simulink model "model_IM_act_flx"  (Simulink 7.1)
settings: Solver=ode45  StartTime=0.0  StopTime=10.0  RelTol=1e-3

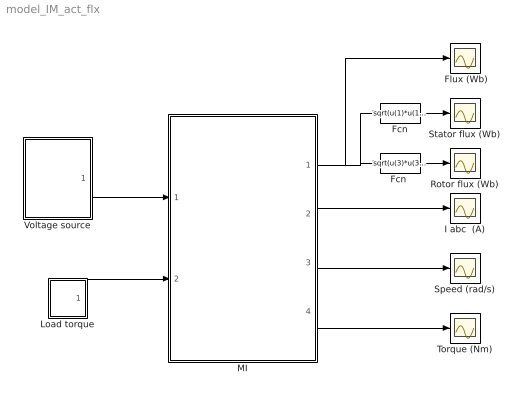
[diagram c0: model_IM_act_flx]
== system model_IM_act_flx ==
  " Flux (Wb)" : Scope
  Fcn : Fcn  Expr=sqrt(u(1)*u(1)+u(2)*u(2))
  "Fcn " : Fcn  Expr=sqrt(u(3)*u(3)+u(4)*u(4))
  I abc  (A) : Scope
  Load torque : Subsystem  mask(Repeating table){}
      mask help: Repeating table. Enter values of time and output for first cycle.
      mask init:
      | period = max(@1); t = @1; y = @2;
  MI : Subsystem  mask(Parameter of induction machine){p=2, Rs=0.3, Rr=0.25, Ls=0.0415, Lr=0.0412, Lm=0.0403, J=0.1, B=0.02}
      mask prompts: p "Poles pairs"; J "Inertial moment"; B "Friction coeficient"
      mask help: The induction machine model in dq frame
      mask init:
      | sigma=1-Lm^2/(Ls*Lr);
      | a11=Rs/(sigma*Ls);
      | a12=Rs*(1-sigma)/(sigma*Lm);
      | a21=Rr*(1-sigma)/(sigma*Lm);
      | a22=Rr/(sigma*Lr);
      | c1=1/(sigma*Ls) ;
      | c2=(sigma-1)/(sigma*Lm);
  Rotor flux (Wb) : Scope
  Speed (rad/s) : Scope
  Stator flux (Wb) : Scope
  Torque (Nm) : Scope
  Voltage source : Subsystem  mask{Vf=220, f1=50}
      mask prompts: Vf "Vf -phase rms value (V)"; f1 "f1 (Hz)"
      mask init:
      | Vm=sqrt(2)*Vf;
      | w1=2*pi*f1;
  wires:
  Fcn/1 -> Stator flux (Wb)/1
  "Fcn "/1 -> Rotor flux (Wb)/1
  MI/1(flux) -> "Fcn "/1, Fcn/1, " Flux (Wb)"/1
  MI/3(w) -> Speed (rad/s)/1
  MI/2("i abc ") -> I abc  (A)/1
  MI/4(Te) -> Torque (Nm)/1
  Voltage source/1(Vabc) -> MI/1(V abc)
  Load torque/1(out_1) -> MI/2(Tload)

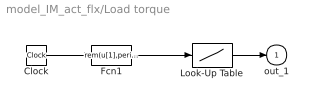
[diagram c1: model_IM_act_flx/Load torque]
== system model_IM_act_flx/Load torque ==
  Clock : Clock
  Fcn1 : Fcn  Expr=rem(u[1],period)
  Look-Up Table : Lookup  InputValues=t  Table=y  OutDataType=sfix(16)  OutScaling=2^0
  out_1 : Outport
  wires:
  Look-Up Table/1 -> out_1/1
  Clock/1 -> Fcn1/1
  Fcn1/1 -> Look-Up Table/1

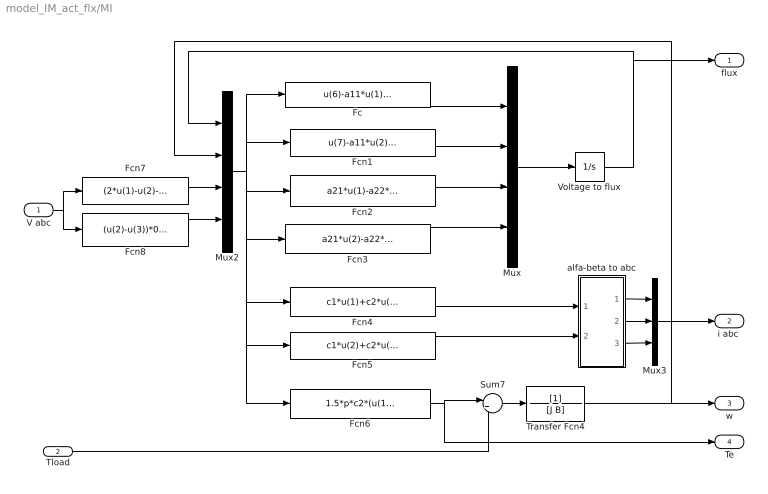
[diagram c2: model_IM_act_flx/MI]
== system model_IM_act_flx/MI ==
  V abc : Inport  OutDataType=sfix(16)  OutScaling=2^0
  Tload : Inport  Port=2  OutDataType=sfix(16)  OutScaling=2^0
  Fc : Fcn  Expr=u(6)-a11*u(1)+a12*u(3)
  Fcn1 : Fcn  Expr=u(7)-a11*u(2)+a12*u(4)
  Fcn2 : Fcn  Expr=a21*u(1)-a22*u(3)-p*u(5)*u(4)
  Fcn3 : Fcn  Expr=a21*u(2)-a22*u(4)+p*u(5)*u(3)
  Fcn4 : Fcn  Expr=c1*u(1)+c2*u(3)
  Fcn5 : Fcn  Expr=c1*u(2)+c2*u(4)
  Fcn6 : Fcn  Expr=1.5*p*c2*(u(1)*u(4)-u(2)*u(3))
  Fcn7 : Fcn  Expr=(2*u(1)-u(2)-u(3))/3
  Fcn8 : Fcn  Expr=(u(2)-u(3))*0.5773502
  Mux : Mux
  Mux2 : Mux
  Mux3 : Mux  Inputs=3
  Sum7 : Sum  Inputs=|+-  OutDataType=sfix(16)  OutScaling=2^0
  Transfer Fcn4 : TransferFcn  Denominator=[J B]
  Voltage to flux : Integrator
  alfa-beta to abc : Subsystem
  flux : Outport
  "i abc " : Outport  Port=2
  w : Outport  Port=3
  Te : Outport  Port=4
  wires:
  Fc/1 -> Mux/1
  Fcn1/1 -> Mux/2
  Fcn2/1 -> Mux/3
  Fcn3/1 -> Mux/4
  Mux2/1 -> Fc/1, Fcn1/1, Fcn2/1, Fcn3/1, Fcn4/1, Fcn6/1, Fcn5/1
  Mux/1 -> Voltage to flux/1
  Voltage to flux/1 -> flux/1, Mux2/1
  Sum7/1 -> Transfer Fcn4/1
  Tload/1 -> Sum7/2
  Fcn6/1 -> Sum7/1, Te/1
  Fcn5/1 -> alfa-beta to abc/2(in_2)
  Transfer Fcn4/1 -> w/1, Mux2/2
  Fcn7/1 -> Mux2/3
  Fcn8/1 -> Mux2/4
  V abc/1 -> Fcn8/1, Fcn7/1
  Mux3/1 -> "i abc "/1
  alfa-beta to abc/1(out_1) -> Mux3/1
  alfa-beta to abc/2(out_2) -> Mux3/2
  alfa-beta to abc/3(out_3) -> Mux3/3
  Fcn4/1 -> alfa-beta to abc/1(in_1)

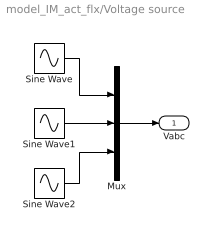
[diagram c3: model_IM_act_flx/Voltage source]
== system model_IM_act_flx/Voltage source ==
  Mux : Mux  Inputs=3
  Sine Wave : Sin  Amplitude=Vm  Frequency=w1  SampleTime=0
  Sine Wave1 : Sin  Amplitude=Vm  Frequency=w1  Phase=-2*pi/3  SampleTime=0
  Sine Wave2 : Sin  Amplitude=Vm  Frequency=w1  Phase=2*pi/3  SampleTime=0
  Vabc : Outport
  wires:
  Sine Wave/1 -> Mux/1
  Sine Wave1/1 -> Mux/2
  Sine Wave2/1 -> Mux/3
  Mux/1 -> Vabc/1

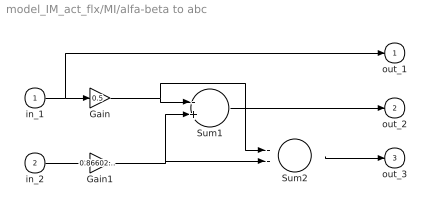
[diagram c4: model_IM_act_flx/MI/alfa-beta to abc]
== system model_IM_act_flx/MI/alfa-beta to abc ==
  in_1 : Inport  OutDataType=sfix(16)  OutScaling=2^0
  in_2 : Inport  Port=2  OutDataType=sfix(16)  OutScaling=2^0
  Gain : Gain  Gain=0.5  ParameterDataType=sfix(16)  ParameterScaling=2^0  OutDataType=sfix(16)  OutScaling=2^0
  Gain1 : Gain  Gain=0.8660254  ParameterDataType=sfix(16)  ParameterScaling=2^0  OutDataType=sfix(16)  OutScaling=2^0
  Sum1 : Sum  Inputs=-+  OutDataType=sfix(16)  OutScaling=2^0
  Sum2 : Sum  Inputs=--  OutDataType=sfix(16)  OutScaling=2^0
  out_1 : Outport  InitialOutput=0
  out_2 : Outport  Port=2  InitialOutput=0
  out_3 : Outport  Port=3  InitialOutput=0
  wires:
  Gain1/1 -> Sum2/2, Sum1/2
  in_2/1 -> Gain1/1
  in_1/1 -> out_1/1, Gain/1
  Gain/1 -> Sum2/1, Sum1/1
  Sum2/1 -> out_3/1
  Sum1/1 -> out_2/1
